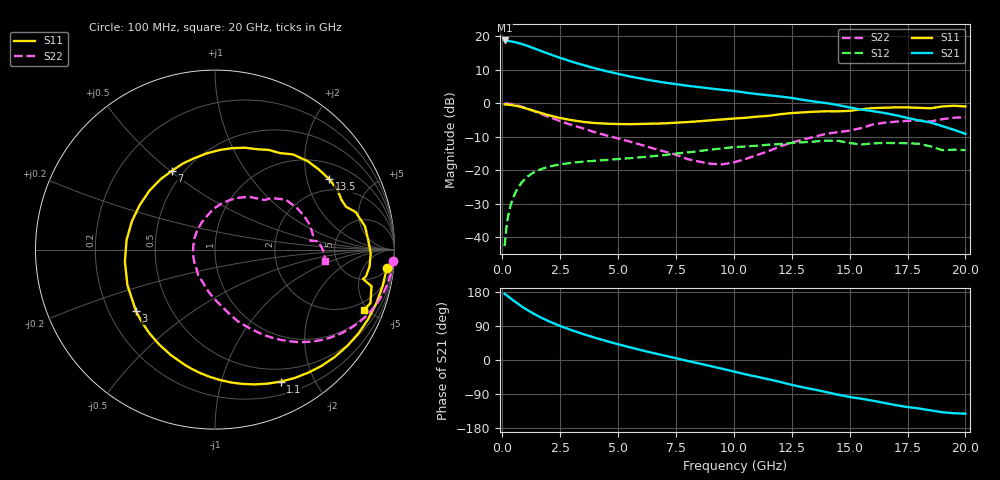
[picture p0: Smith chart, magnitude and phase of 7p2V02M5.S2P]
! Infineon Technologies  Discrete & RF Semiconductors
! bfp620
! VCE =  2.0 V,  IC =  2.5 mA
! Common Emitter S-Parameters:  Sep 2002
# GHz  S  MA  R  50
!  f  S11  S21  S12  S22
! GHz  MAG  ANG  MAG  ANG  MAG  ANG  MAG  ANG
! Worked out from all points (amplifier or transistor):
!   59 points, 100 MHz to 20 GHz, reference 50 ohm
!   highest |S21| = 18.7 dB at 100 MHz (marker M1)
!   |S21| within 3 dB of that: start of sweep to 1.621 GHz
!   unconditionally stable (mu >= 1): 5.516 GHz to 13.44 GHz; 14.2 GHz to 15.64 GHz; 17.48 GHz to end of sweep
!   at 1 GHz: K = 0.19, MSG = 19.9 dB, |S12| = -22.5 dB
!   at 5.5 GHz: K = 1.00, MSG = 12.2 dB, |S12| = -16.4 dB
!   at 20 GHz: K = 1.35, MAG = -1.1 dB, |S12| = -14.0 dB
!   S11 on the Smith chart (normalised r, x): 100 MHz: 6, -16; 1.1 GHz: 0.34, -1.56; 3 GHz: 0.31, -0.31; 7 GHz: 0.43, +0.51; 13.5 GHz: 1.53, +2.73; 20 GHz: 1.38, -4.71
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0.1  0.9626 -6.2  8.617 174.6  0.0074 80.3  0.9955 -3.6
0.2  0.9559 -12.2  8.524 170.2  0.0164 81.9  0.9905 -7.2
0.3  0.9476 -18.3  8.423 165.5  0.0251 79.6  0.9818 -10.8
0.6  0.9118 -36.1  8.039 151.7  0.049 69.7  0.937 -21.0
0.8  0.8788 -47.5  7.701 143.1  0.0631 63.1  0.8959 -27.2
1.1  0.8217 -63.5  7.112 131.3  0.0808 54.1  0.8257 -35.5
1.5  0.7456 -83.1  6.322 117.4  0.0983 44.1  0.7309 -44.7
2  0.6638 -104.7  5.458 102.6  0.1126 34.4  0.6274 -53.5
2.4  0.6134 -120.5  4.869 92.3  0.1207 28.5  0.5581 -59.3
3  0.5583 -142.0  4.164 78.5  0.1293 21.3  0.474 -66.7
3.5  0.5266 -157.9  3.704 68.3  0.1348 16.5  0.4207 -72.2
4  0.5064 -172.5  3.315 58.8  0.1386 12.4  0.3694 -77.2
5  0.4893 160.8  2.737 41.5  0.147 6.5  0.2986 -86.3
6  0.4911 138.3  2.33 26.0  0.1567 1.5  0.2396 -98.2
7  0.5005 118.6  2.03 11.8  0.169 -3.0  0.1907 -112.1
8.5  0.5382 94.7  1.737 -9.2  0.1937 -11.6  0.1347 -149.5
10.5  0.6064 67.3  1.442 -37.8  0.2267 -27.8  0.1472 132.0
12  0.6855 50.7  1.26 -57.9  0.2458 -39.2  0.2267 92.3
13.5  0.7475 31.8  1.055 -78.3  0.2685 -53.2  0.3185 65.2
15  0.7681 18.1  0.866 -97.5  0.2559 -72.6  0.3901 45.1
17  0.868 -1.4  0.662 -119.2  0.2542 -84.6  0.5305 20.7
20  0.8953 -22.2  0.35 -141.6  0.2 -104.2  0.6173 -5.9
